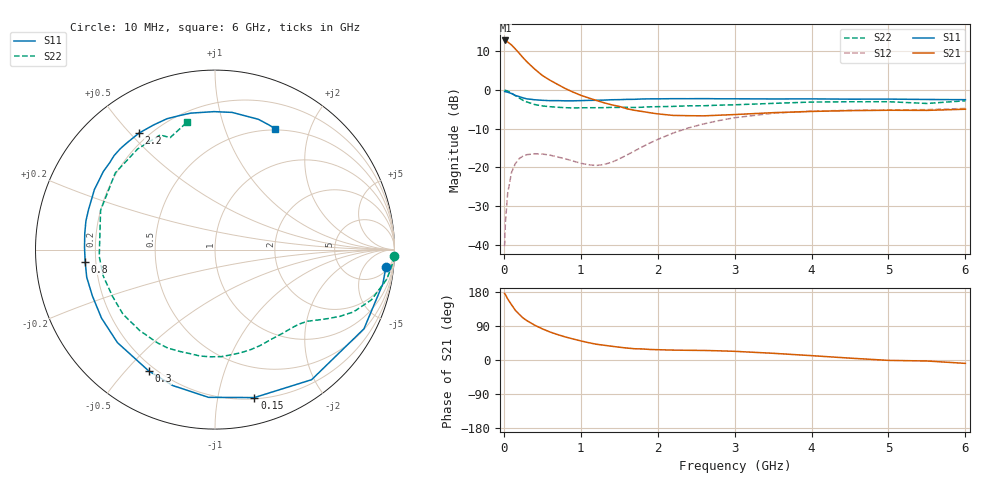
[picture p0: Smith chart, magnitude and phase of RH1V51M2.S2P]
! SIEMENS Small Signal Semiconductors
! BFR106
! Si NPN RF Bipolar Junction Transistor in SOT23
! VCE = 1.5 V  IC = 1.2 mA
! Common Emitter S-Parameters:  August  1996
# GHz  S  MA  R  50
!  f  S11  S21  S12  S22
! GHz  MAG  ANG  MAG  ANG  MAG  ANG  MAG  ANG
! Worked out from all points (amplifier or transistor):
!   36 points, 10 MHz to 6 GHz, reference 50 ohm
!   highest |S21| = 12.8 dB at 20 MHz (marker M1)
!   |S21| within 3 dB of that: start of sweep to 185.7 MHz
!   unconditionally stable (mu >= 1): 826.5 MHz to end of sweep
!   at 250 MHz: K = 0.29, MSG = 12.7 dB, |S12| = -17.0 dB
!   at 1.4 GHz: K = 1.47, MAG = 3.4 dB, |S12| = -18.7 dB
!   at 6 GHz: K = 1.02, MAG = -1.0 dB, |S12| = -4.7 dB
!   S11 on the Smith chart (normalised r, x): 10 MHz: 7, -17; 150 MHz: 0.21, -1.28; 300 MHz: 0.17, -0.58; 800 MHz: 0.16, -0.05; 2.2 GHz: 0.16, +0.53; 6 GHz: 0.49, +1.51
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0.01  0.9578 -5.7  4.36 175.7  0.0096 89.0  0.9993 -2.1
0.02  0.9543 -11.6  4.386 172.7  0.0192 83.9  0.9945 -4.0
0.05  0.94 -28.0  4.191 161.2  0.0466 73.6  0.9718 -9.7
0.1  0.9029 -53.4  3.834 145.8  0.0862 60.3  0.9154 -17.8
0.15  0.8531 -75.1  3.402 131.1  0.1125 48.1  0.8465 -24.2
0.2  0.824 -92.5  2.993 120.6  0.1302 39.9  0.7895 -28.1
0.25  0.7931 -107.3  2.624 110.9  0.1407 32.9  0.7374 -31.4
0.3  0.7701 -118.7  2.324 103.8  0.1463 28.1  0.7026 -33.8
0.4  0.751 -136.4  1.873 92.0  0.1504 20.6  0.6514 -37.8
0.5  0.7386 -148.9  1.548 82.2  0.1492 15.8  0.6249 -41.7
0.6  0.7303 -159.4  1.342 73.9  0.1443 13.1  0.6102 -45.9
0.8  0.7266 -174.7  1.047 60.8  0.1295 12.6  0.5923 -55.2
1.1  0.7368 167.4  0.794 45.8  0.1083 23.9  0.5917 -70.5
1.3  0.7429 157.6  0.687 39.0  0.1093 39.4  0.593 -81.3
1.6  0.7592 145.0  0.574 31.5  0.1449 57.9  0.5987 -98.1
2.2  0.7749 123.1  0.471 26.1  0.2782 60.1  0.6157 -132.8
2.8  0.7724 104.8  0.474 24.2  0.4045 46.7  0.6397 -166.7
3.5  0.7687 90.4  0.511 17.7  0.5022 29.7  0.6738 161.1
4.5  0.7639 77.0  0.543 4.9  0.5481 10.0  0.7071 127.6
5  0.7652 71.6  0.549 -1.0  0.5539 2.9  0.708 115.6
5.5  0.7568 66.6  0.547 -2.6  0.5594 -0.3  0.6721 111.8
6  0.7521 63.4  0.566 -8.9  0.5798 -7.6  0.728 102.2
